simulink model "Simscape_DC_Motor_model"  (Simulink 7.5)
settings: Solver=ode45  StartTime=0.0  StopTime=40  RelTol=1e-3
PreLoadFcn:
  | L=7;
  | R=10;
  | K=12/4000;
  | I=0.0002;
  | k1 = 12;
  | k2 = 12/4000;
  | k3=12;
  | k4=-12;
  | k5=-1.9;
  | k6=1;
  | 
  | 
  | I_init=0.0002;I_min=0.0001; I_max=0.001;
  | K_init=12/4000;K_min=0.0002; K_max=0.003;
  | L_init=7; L_min=0; L_max=400;
  | R_init=10; R_min=0; R_max=400;
  | K2_init=12/4000; K2_min=0.0002; K2_max=0.003;
libraries: fl_lib x10, nesl_utility x4

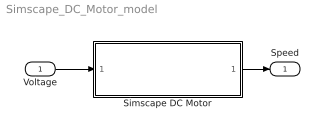
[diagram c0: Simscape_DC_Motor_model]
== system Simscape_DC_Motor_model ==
  Voltage : Inport  OutDataType=fixdt(1, 16)  OutScaling=2^0
  Simscape DC Motor : Subsystem
  Speed : Outport  OutDataType=fixdt(1, 16)  OutScaling=2^0
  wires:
  Voltage/1 -> Simscape DC Motor/1(Voltage)
  Simscape DC Motor/1(Speed) -> Speed/1

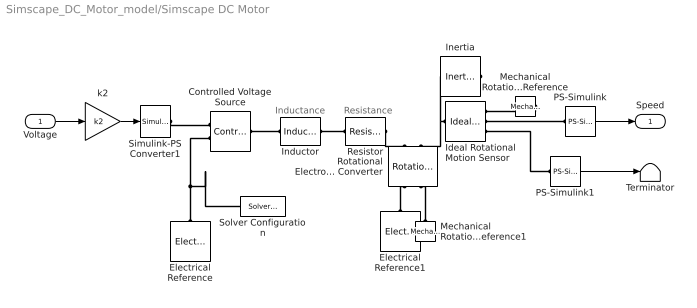
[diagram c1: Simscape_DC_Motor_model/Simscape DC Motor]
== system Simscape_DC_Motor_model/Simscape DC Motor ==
  note: Resistance
  note: Inductance
  Voltage : Inport  OutDataType=fixdt(1, 16)  OutScaling=2^0
  Controlled Voltage Source : fl_lib/Electrical/Electrical Sources/Controlled Voltage Source  DialogController=NetworkEngine.DynNeDlgSource  SystemSampleTime=-1  i_Log=off  v_Log=off  LocalVarNames=|i|v  LocalVarDescs=|i|v  LocalVarLogging=[0 0]
  Electrical Reference : fl_lib/Electrical/Electrical Elements/Electrical Reference  DialogController=NetworkEngine.DynNeDlgSource  SystemSampleTime=-1  i_Log=off  LocalVarNames=|i  LocalVarDescs=|i  LocalVarLogging=0
  Electrical Reference1 : fl_lib/Electrical/Electrical Elements/Electrical Reference  DialogController=NetworkEngine.DynNeDlgSource  SystemSampleTime=-1  i_Log=off  LocalVarNames=|i  LocalVarDescs=|i  LocalVarLogging=0
  Ideal Rotational Motion Sensor : fl_lib/Mechanical/Mechanical Sensors/Ideal Rotational Motion Sensor  DialogController=NetworkEngine.DynNeDlgSource  SystemSampleTime=-1  offset=0 deg  w_Log=off  t_Log=off  phi_Log=off  LocalVarNames=|w|t|phi  LocalVarDescs=|w|t|phi  LocalVarLogging=[]
  Inductor : fl_lib/Electrical/Electrical Elements/Inductor  DialogController=NetworkEngine.DynNeDlgSource  SystemSampleTime=-1  l=L mH  i0=0 A  r=0 Ohm  g=1e-9 1/Ohm  i_Log=off  v_Log=off  i_L_Log=off  LocalVarNames=|i|v|i_L  LocalVarDescs=|i|v|Internal variable for current through inductor term  LocalVarLogging=[0 0 0]
  Inertia : fl_lib/Mechanical/Rotational Elements/Inertia  DialogController=NetworkEngine.DynNeDlgSource  SystemSampleTime=-1  inertia=I kg*m^2  initial_velocity=0 rad/s  t_Log=off  LocalVarNames=|t  LocalVarDescs=|t  LocalVarLogging=0
  Mechanical Rotational Reference : fl_lib/Mechanical/Rotational Elements/Mechanical Rotational Reference  DialogController=NetworkEngine.DynNeDlgSource  SystemSampleTime=-1  t_Log=off  LocalVarNames=|t  LocalVarDescs=|t  LocalVarLogging=[]
  Mechanical Rotational Reference1 : fl_lib/Mechanical/Rotational Elements/Mechanical Rotational Reference  DialogController=NetworkEngine.DynNeDlgSource  SystemSampleTime=-1  t_Log=off  LocalVarNames=|t  LocalVarDescs=|t  LocalVarLogging=[]
  PS-Simulink : nesl_utility/PS-Simulink Converter  DialogController=NetworkEngine.DynNeUtilDlgSource  SystemSampleTime=-1  PhysicalDomain=network_engine_domain  LeftPortType=input  RightPortType=output  SubClassName=ps_output  Unit=rpm  AffineConversion=off
  PS-Simulink1 : nesl_utility/PS-Simulink Converter  DialogController=NetworkEngine.DynNeUtilDlgSource  SystemSampleTime=-1  PhysicalDomain=network_engine_domain  LeftPortType=input  RightPortType=output  SubClassName=ps_output  Unit=1  AffineConversion=off
  Resistor : fl_lib/Electrical/Electrical Elements/Resistor  DialogController=NetworkEngine.DynNeDlgSource  SystemSampleTime=-1  R=R Ohm  i_Log=off  v_Log=off  LocalVarNames=|i|v  LocalVarDescs=|i|v  LocalVarLogging=[0 0]
  Rotational Electromechanical Converter : fl_lib/Electrical/Electrical Elements/Rotational Electromechanical Converter  DialogController=NetworkEngine.DynNeDlgSource  SystemSampleTime=-1  K=K V/rpm  i_Log=off  v_Log=off  t_Log=off  w_Log=off  LocalVarNames=|i|v|t|w  LocalVarDescs=|i|v|t|w  LocalVarLogging=[0 0 0 0]
  Simulink-PS Converter1 : nesl_utility/Simulink-PS Converter  DialogController=NetworkEngine.DynNeUtilDlgSource  SystemSampleTime=-1  PhysicalDomain=network_engine_domain  LeftPortType=input  RightPortType=output  SubClassName=ps_input  Unit=V  AffineConversion=off  InputFilterTimeConstant=.001  UdotUserProvided=0
  Solver Configuration : nesl_utility/Solver Configuration  DialogController=NetworkEngine.DynNeUtilDlgSource  SystemSampleTime=-1  PhysicalDomain=network_engine_domain  LeftPortType=input  RightPortType=generic  SubClassName=solver  Accelerate=off  Profile=off  ResidualTolerance=1e-9  MaxNonlinIter=3  MaxModeIter=2  DoFixedCost=off  UseLocalSampling=off  DoDC=off  LinearAlgebra=Sparse  LocalSolverSampleTime=.001  LocalSolverChoice=NE_BACKWARD_EULER_ADVANCER  UseLocalSolver=off
  Terminator : Terminator
  k2 : Gain  Gain=k2  ParameterDataType=fixdt(1, 16)  ParameterScaling=2^0  OutDataType=fixdt(1, 16)  OutScaling=2^0
  Speed : Outport  OutDataType=fixdt(1, 16)  OutScaling=2^0
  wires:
  Voltage/1 -> k2/1
  PS-Simulink/1 -> Speed/1
  k2/1 -> Simulink-PS Converter1/1
  PS-Simulink1/1 -> Terminator/1
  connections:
  Controlled Voltage Source/LConn1 -- Inductor/LConn1
  Simulink-PS Converter1/RConn1 -- Controlled Voltage Source/RConn1
  Electrical Reference/LConn1 -- Controlled Voltage Source/RConn2 -- Solver Configuration/RConn1
  Electrical Reference1/LConn1 -- Rotational Electromechanical Converter/RConn1
  Ideal Rotational Motion Sensor/LConn1 -- Inertia/LConn1 -- Rotational Electromechanical Converter/LConn2
  Mechanical Rotational Reference/LConn1 -- Ideal Rotational Motion Sensor/RConn1
  PS-Simulink/LConn1 -- Ideal Rotational Motion Sensor/RConn2
  PS-Simulink1/LConn1 -- Ideal Rotational Motion Sensor/RConn3
  Inductor/RConn1 -- Resistor/LConn1
  Mechanical Rotational Reference1/LConn1 -- Rotational Electromechanical Converter/RConn2
  Resistor/RConn1 -- Rotational Electromechanical Converter/LConn1
